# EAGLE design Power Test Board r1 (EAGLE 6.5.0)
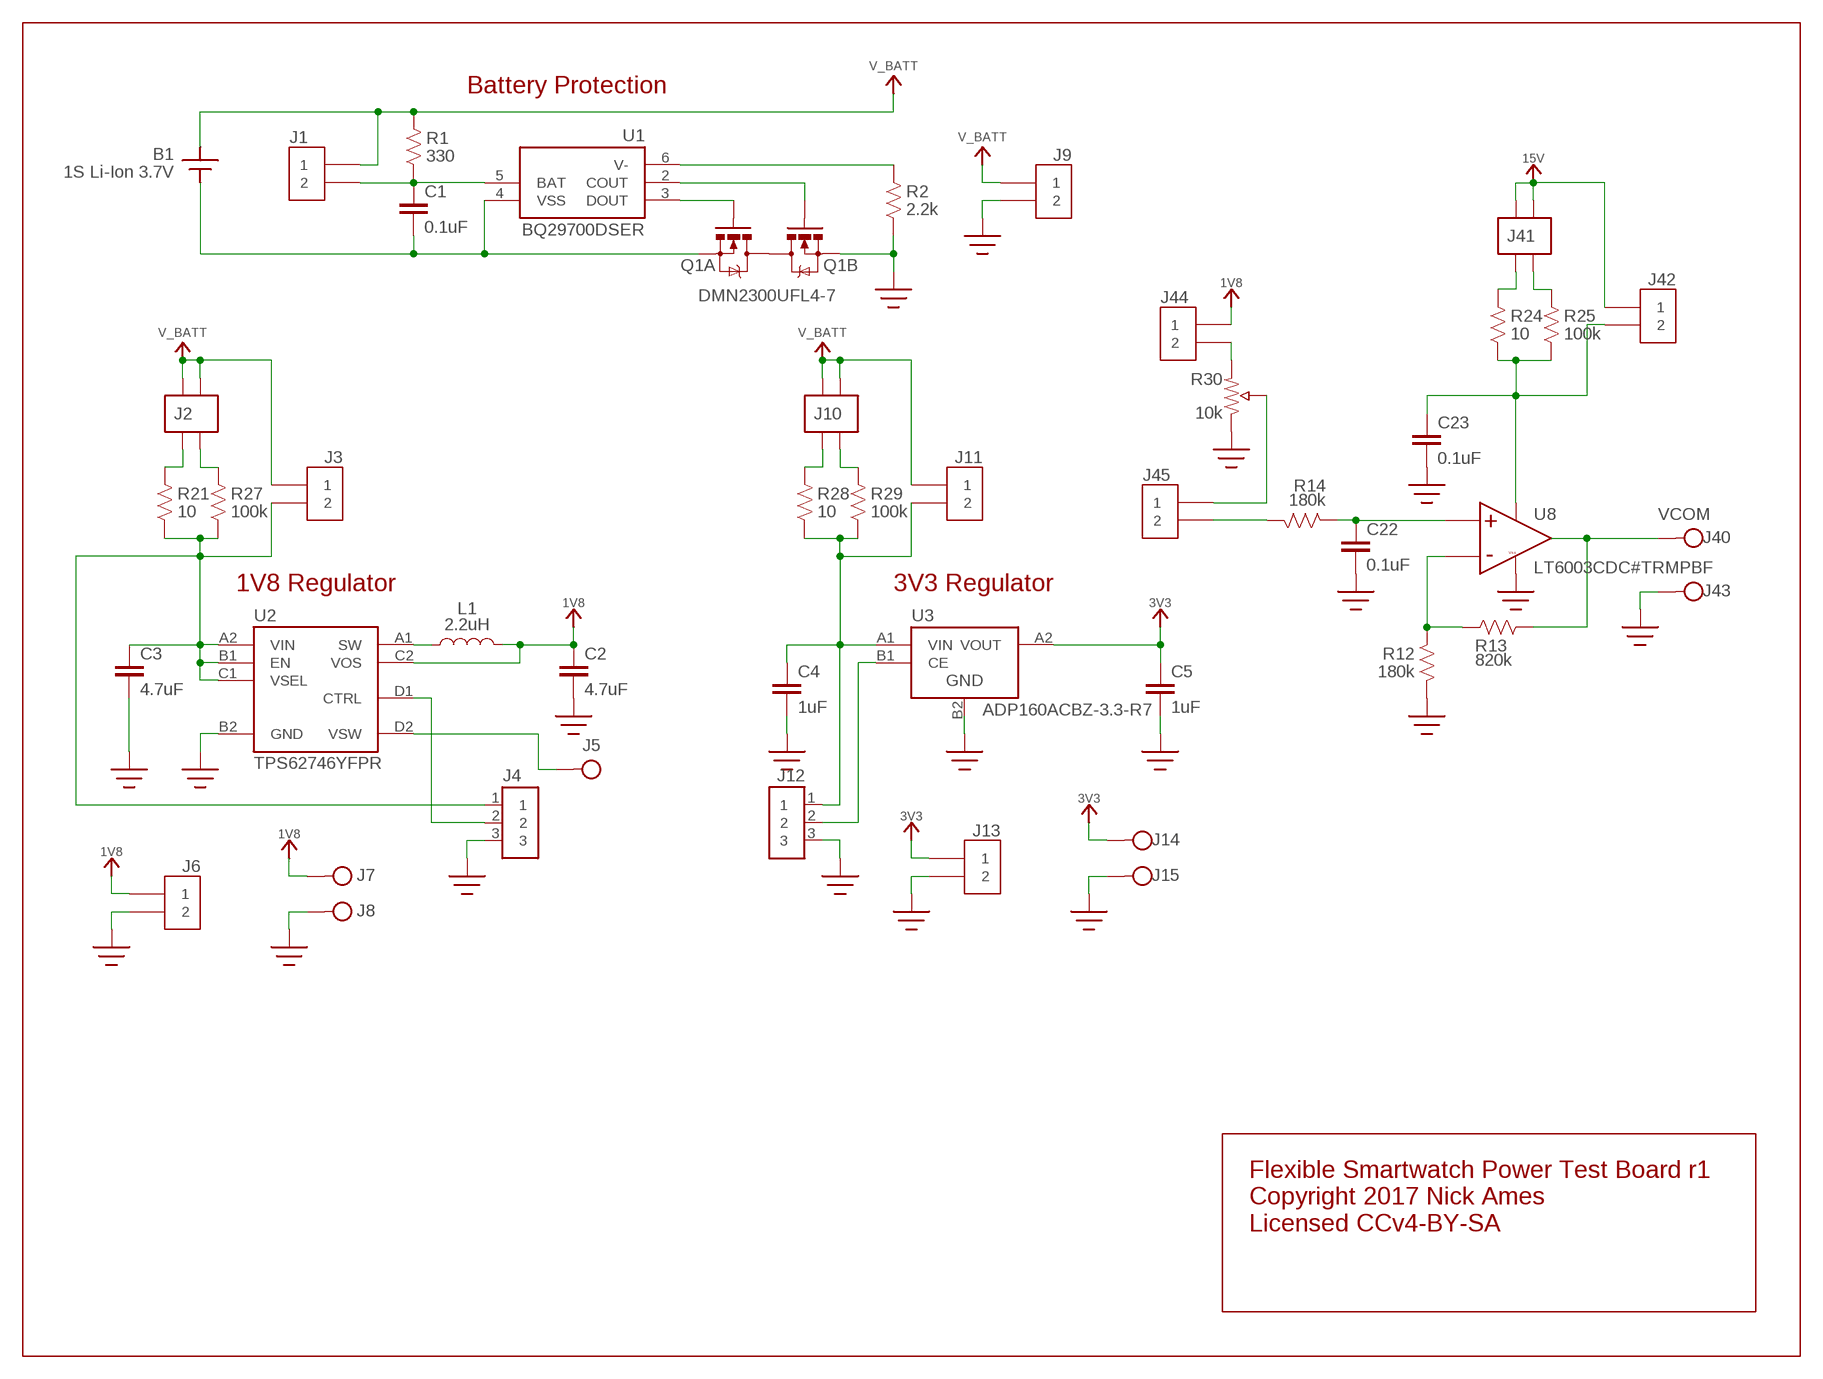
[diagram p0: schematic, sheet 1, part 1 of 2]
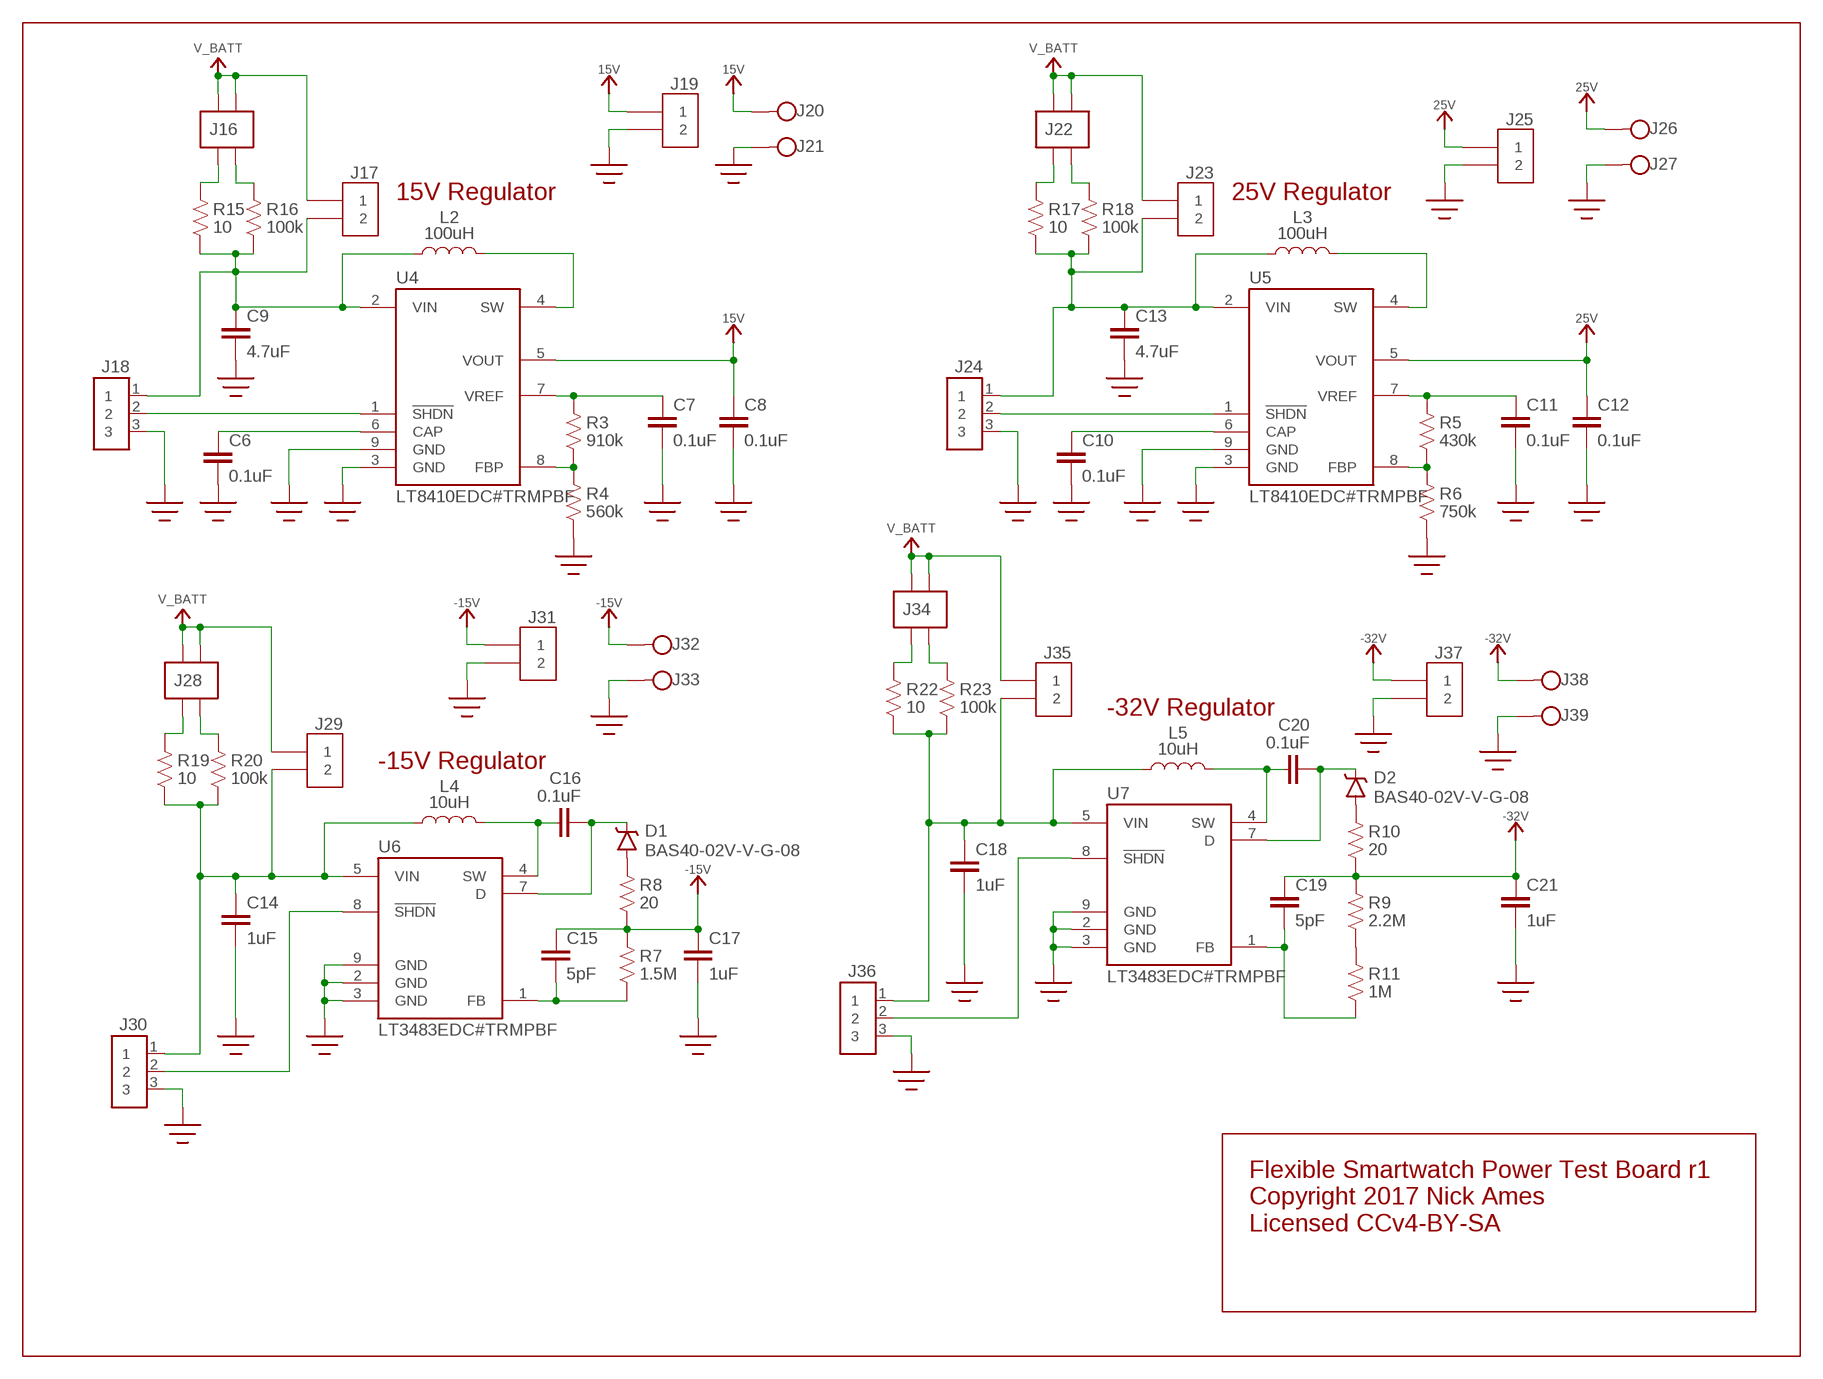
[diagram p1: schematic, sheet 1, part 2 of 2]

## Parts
B1  1S Li-Ion 3.7V  BATTERY-1CELLWIRE_TERMINAL_PTH  [BATTERY-WIRETERM]
C1  0.1uF  CAP201  [0201]
C2  4.7uF  CAP201  [0201]
C3  4.7uF  CAP201  [0201]
C4  1uF  CAP201  [0201]
C5  1uF  CAP201  [0201]
C6  0.1uF  CAP201  [0201]
C7  0.1uF  CAP201  [0201]
C8  0.1uF  CAP201  [0201]
C9  4.7uF  CAP201  [0201]
C10  0.1uF  CAP201  [0201]
C11  0.1uF  CAP201  [0201]
C12  0.1uF  CAP201  [0201]
C13  4.7uF  CAP201  [0201]
C14  1uF  CAP201  [0201]
C15  5pF  CAP201  [0201]
C16  0.1uF  CAP201  [0201]
C17  1uF  CAP402  [0402]
C18  1uF  CAP201  [0201]
C19  5pF  CAP201  [0201]
C20  0.1uF  CAP201  [0201]
C21  1uF  CAP402  [0402]
C22  0.1uF  CAP201  [0201]
C23  0.1uF  CAP201  [0201]
D1  BAS40-02V-V-G-08  DIODE-SCHOTTKYSOD-523  [SOD-523]
D2  BAS40-02V-V-G-08  DIODE-SCHOTTKYSOD-523  [SOD-523]
J1  HEADER-02HEADER-02  [HEADER-02]
J2  HEADER-02X02  [HEADER-02X02]
J3  HEADER-02HEADER-02  [HEADER-02]
J4  HEADER-03PTH  [HEADER-03]
J5  TESTPOINTPTH  [TESTPOINT-1-PTH]
J6  HEADER-02HEADER-02  [HEADER-02]
J7  TESTPOINTPTH  [TESTPOINT-1-PTH]
J8  TESTPOINTPTH  [TESTPOINT-1-PTH]
J9  HEADER-02HEADER-02  [HEADER-02]
J10  HEADER-02X02  [HEADER-02X02]
J11  HEADER-02HEADER-02  [HEADER-02]
J12  HEADER-03PTH  [HEADER-03]
J13  HEADER-02HEADER-02  [HEADER-02]
J14  TESTPOINTPTH  [TESTPOINT-1-PTH]
J15  TESTPOINTPTH  [TESTPOINT-1-PTH]
J16  HEADER-02X02  [HEADER-02X02]
J17  HEADER-02HEADER-02  [HEADER-02]
J18  HEADER-03PTH  [HEADER-03]
J19  HEADER-02HEADER-02  [HEADER-02]
J20  TESTPOINTPTH  [TESTPOINT-1-PTH]
J21  TESTPOINTPTH  [TESTPOINT-1-PTH]
J22  HEADER-02X02  [HEADER-02X02]
J23  HEADER-02HEADER-02  [HEADER-02]
J24  HEADER-03PTH  [HEADER-03]
J25  HEADER-02HEADER-02  [HEADER-02]
J26  TESTPOINTPTH  [TESTPOINT-1-PTH]
J27  TESTPOINTPTH  [TESTPOINT-1-PTH]
J28  HEADER-02X02  [HEADER-02X02]
J29  HEADER-02HEADER-02  [HEADER-02]
J30  HEADER-03PTH  [HEADER-03]
J31  HEADER-02HEADER-02  [HEADER-02]
J32  TESTPOINTPTH  [TESTPOINT-1-PTH]
J33  TESTPOINTPTH  [TESTPOINT-1-PTH]
J34  HEADER-02X02  [HEADER-02X02]
J35  HEADER-02HEADER-02  [HEADER-02]
J36  HEADER-03PTH  [HEADER-03]
J37  HEADER-02HEADER-02  [HEADER-02]
J38  TESTPOINTPTH  [TESTPOINT-1-PTH]
J39  TESTPOINTPTH  [TESTPOINT-1-PTH]
J40  TESTPOINTPTH  [TESTPOINT-1-PTH]
J41  HEADER-02X02  [HEADER-02X02]
J42  HEADER-02HEADER-02  [HEADER-02]
J43  TESTPOINTPTH  [TESTPOINT-1-PTH]
J44  HEADER-02HEADER-02  [HEADER-02]
J45  HEADER-02HEADER-02  [HEADER-02]
L1  2.2uH  INDUCTOR603  [0603-RES]
L2  100uH  INDUCTOR805  [0805-IND]
L3  100uH  INDUCTOR805  [0805-IND]
L4  10uH  INDUCTORMDKK2020  [TY_MDKK2020]
L5  10uH  INDUCTORMDKK2020  [TY_MDKK2020]
Q1  DMN2300UFL4-7  MOSFET-N-DUALDFN  [DFN1310-6]
R1  330  RESISTOR201  [0201]
R2  2.2k  RESISTOR201  [0201]
R3  910k  RESISTOR201  [0201]
R4  560k  RESISTOR201  [0201]
R5  430k  RESISTOR201  [0201]
R6  750k  RESISTOR201  [0201]
R7  1.5M  RESISTOR201  [0201]
R8  20  RESISTOR201  [0201]
R9  2.2M  RESISTOR201  [0201]
R10  20  RESISTOR201  [0201]
R11  1M  RESISTOR201  [0201]
R12  180k  RESISTOR201  [0201]
R13  820k  RESISTOR201  [0201]
R14  180k  RESISTOR201  [0201]
R15  10  RESISTOR0603-RES  [0603-RES]
R16  100k  RESISTOR0603-RES  [0603-RES]
R17  10  RESISTOR0603-RES  [0603-RES]
R18  100k  RESISTOR0603-RES  [0603-RES]
R19  10  RESISTOR0603-RES  [0603-RES]
R20  100k  RESISTOR0603-RES  [0603-RES]
R21  10  RESISTOR0603-RES  [0603-RES]
R22  10  RESISTOR0603-RES  [0603-RES]
R23  100k  RESISTOR0603-RES  [0603-RES]
R24  10  RESISTOR0603-RES  [0603-RES]
R25  100k  RESISTOR0603-RES  [0603-RES]
R27  100k  RESISTOR0603-RES  [0603-RES]
R28  10  RESISTOR0603-RES  [0603-RES]
R29  100k  RESISTOR0603-RES  [0603-RES]
R30  10k  POTPVZA3  [PVZ3A]
U1  BQ29700DSER  TI-BQ29700_BATTERY_PROTECTOR  [6-SON_TI_DSE]
U2  TPS62746YFPR  TI-TPS62746_VREG_BUCK_VSWITCH  [8-XBGA_TI_YFP]
U3  ADP160ACBZ-3.3-R7  AD_ADP160CBZ  [WLCSP-4-.5]
U4  LT8410EDC#TRMPBF  LT-LT8410_VREG_BOOST  [8-DFN_LT_DC]
U5  LT8410EDC#TRMPBF  LT-LT8410_VREG_BOOST  [8-DFN_LT_DC]
U6  LT3483EDC#TRMPBF  LT-LT3483_VREG_INVERT  [8-DFN_LT_DC]
U7  LT3483EDC#TRMPBF  LT-LT3483_VREG_INVERT  [8-DFN_LT_DC]
U8  LT6003CDC#TRMPBF  OPAMPLT6003  [DFN-4_LT_DC]

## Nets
1V8: C2.P$1 J6.1 J7.1 J44.1 L1.2 U2.C2(VOS)
3V3: C5.P$1 J13.1 J14.1 U3.A2(VOUT)
15V: C8.P$1 J19.1 J20.1 J41.1 J41.4 J42.1 U4.5(VOUT)
25V: C12.P$1 J25.1 J26.1 U5.5(VOUT)
-15V: C15.P$1 C17.1 J31.1 J32.1 R7.P$2 R8.P$1
-32V: C19.P$1 C21.1 J37.1 J38.1 R9.P$2 R10.P$1
GND: C2.P$2 C3.P$2 C4.P$2 C5.P$2 C6.P$2 C7.P$2 C8.P$2 C9.P$2 C10.P$2 C11.P$2 C12.P$2 C13.P$2 C14.P$2 C17.2 C18.P$2 C21.2 C22.P$2 C23.P$2 J4.3 J6.2 J8.1 J9.2 J12.3 J13.2 J15.1 J18.3 J19.2 J21.1 J24.3 J25.2 J27.1 J30.3 J31.2 J33.1 J36.3 J37.2 J39.1 J43.1 Q1.S2(B:S) R2.P$1 R4.P$1 R6.P$1 R12.P$1 R30.1(A) U2.B2(GND) U3.B2(GND) U4.3(GND) U4.9(GND) U5.3(GND) U5.9(GND) U6.2(GND) U6.3(GND) U6.9(GND) U7.2(GND) U7.3(GND) U7.9(GND) U8.5(VSS)
N$1: C1.P$1 J1.2 R1.P$1 U1.5(BAT)
N$2: B1.- C1.P$2 Q1.S1(A:S) U1.4(VSS)
N$3: C3.P$1 J3.2 J4.1 R21.1 R27.1 U2.A2(VIN) U2.B1(EN) U2.C1(VSEL)
N$4: Q1.D1(A:D) Q1.D2(B:D)
N$5: Q1.G1(A:G) U1.3(DOUT)
N$6: Q1.G2(B:G) U1.2(COUT)
N$7: R2.P$2 U1.6(V-)
N$8: L1.1 U2.A1(SW)
N$9: C14.P$1 J29.2 J30.1 L4.1 R19.1 R20.1 U6.5(VIN)
N$10: J12.2 U3.B1(CE)
N$11: C4.P$1 J11.2 J12.1 R28.1 R29.1 U3.A1(VIN)
N$12: J10.3 R28.2
N$13: C6.P$1 U4.6(CAP)
N$14: J18.2 U4.1(!SHDN!)
N$15: C9.P$1 J17.2 J18.1 L2.P$1 R15.1 R16.1 U4.2(VIN)
N$16: C7.P$1 R3.P$2 U4.7(VREF)
N$17: L2.P$2 U4.4(SW)
N$18: R3.P$1 R4.P$2 U4.8(FBP)
N$19: C10.P$1 U5.6(CAP)
N$20: J24.2 U5.1(!SHDN!)
N$21: J30.2 U6.8(!SHDN!)
N$22: C11.P$1 R5.P$2 U5.7(VREF)
N$23: L3.P$2 U5.4(SW)
N$24: R5.P$1 R6.P$2 U5.8(FBP)
N$25: J2.3 R21.2
N$26: J2.2 R27.2
N$27: J10.2 R29.2
N$28: J4.2 U2.D1(CTRL)
N$29: J5.1 U2.D2(VSW)
N$30: J16.3 R15.2
N$31: J16.2 R16.2
N$32: C13.P$1 J23.2 J24.1 L3.P$1 R17.1 R18.1 U5.2(VIN)
N$33: C16.P$1 L4.2 U6.4(SW)
N$34: D1.A R8.P$2
N$35: C16.P$2 D1.C U6.7(D)
N$36: J22.3 R17.2
N$37: J22.2 R18.2
N$38: C23.P$1 J42.2 R24.1 R25.1 U8.4(VDD)
N$39: C15.P$2 R7.P$1 U6.1(FB)
N$40: J36.2 U7.8(!SHDN!)
N$41: C20.P$1 L5.2 U7.4(SW)
N$42: D2.A R10.P$2
N$43: C20.P$2 D2.C U7.7(D)
N$44: C19.P$2 R11.P$1 U7.1(FB)
N$45: J34.3 R22.2
N$46: R9.P$1 R11.P$2
N$47: J28.3 R19.2
N$48: J28.2 R20.2
N$49: J34.2 R23.2
N$50: C18.P$1 J35.2 J36.1 L5.1 R22.1 R23.1 U7.5(VIN)
N$51: J41.3 R24.2
N$52: R12.P$2 R13.P$1 U8.2(-)
N$53: C22.P$1 R14.P$1 U8.1(+)
N$54: J44.2 R30.3(E)
N$55: J41.2 R25.2
N$57: J45.2 R14.P$2
N$58: J45.1 R30.2(S)
V_BATT: B1.+ J1.1 J2.1 J2.4 J3.1 J9.1 J10.1 J10.4 J11.1 J16.1 J16.4 J17.1 J22.1 J22.4 J23.1 J28.1 J28.4 J29.1 J34.1 J34.4 J35.1 R1.P$2
VCOM: J40.1 R13.P$2 U8.3(OUT)

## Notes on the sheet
- Battery Protection
- 15V Regulator | 25V Regulator
- 1V8 Regulator | 3V3 Regulator
- -32V Regulator
- -15V Regulator
- Flexible Smartwatch Power Test Board r1
  Copyright 2017 Nick Ames
  Licensed CCv4-BY-SA
- Flexible Smartwatch Power Test Board r1
  Copyright 2017 Nick Ames
  Licensed CCv4-BY-SA

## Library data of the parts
B1 = NA-lib:BATTERY-1CELL
C1-C23 = NA-lib:CAP: Capacitor
D1 D2 = NA-lib:DIODE-SCHOTTKY
J1 J3 J6 J9 J11 J13 J17 J19 J23 J25 J29 J31 J35 J37 J42 J44 J45 = NA-lib:HEADER-02
J2 J10 J16 J22 J28 J34 J41 = NA-lib:HEADER-02X02
J4 J12 J18 J24 J30 J36 = NA-lib:HEADER-03
J5 J7 J8 J14 J15 J20 J21 J26 J27 J32 J33 J38-J40 J43 = NA-lib:TESTPOINT
L1-L5 = NA-lib:INDUCTOR: Inductors
Q1 = NA-lib:MOSFET-N-DUAL
R1-R25 R27-R29 = NA-lib:RESISTOR: Resistor
R30 = NA-lib:POT
U1 = Project-6p:TI-BQ29700_BATTERY_PROTECTOR
U2 = Project-6p:TI-TPS62746_VREG_BUCK_VSWITCH
U3 = NA-lib:AD_ADP160
U4 U5 = Project-6p:LT-LT8410_VREG_BOOST
U6 U7 = Project-6p:LT-LT3483_VREG_INVERT
U8 = NA-lib:OPAMP

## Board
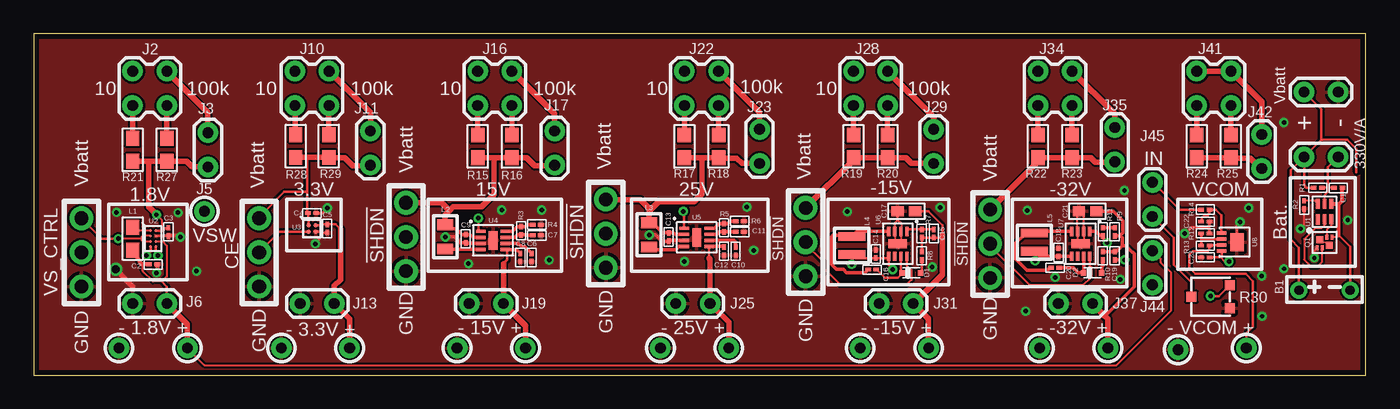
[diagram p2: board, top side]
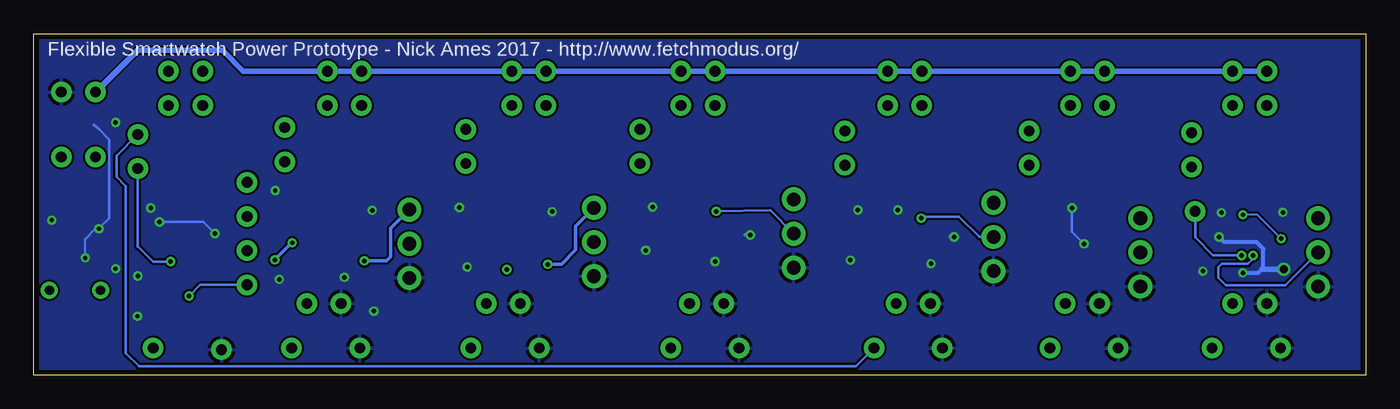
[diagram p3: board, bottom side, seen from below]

Size 99.06 x 25.4 mm. Coordinates in mm from the lower left corner, seen from the top.
Outline: 0,0 99.06,0 99.06,25.4 0,25.4 0,0
Copper layers (1*16): Top 0.0356mm / dielectric 1.5011mm / Bottom 0.0356mm
Design rules "LaenPCBOrder-tented_vias": minimum track width 6mil, minimum drill 13mil, track to track 6mil, track to pad 6mil, pad to pad 6mil, via to via 6mil, smd to smd 6mil, copper to edge 15mil, drill to drill 6mil, minimum pad ring 7mil, minimum via ring 7mil, stop-mask expansion 3mil, vias tented up to drill 25mil, thermal gap 10mil
tRestrict: area 63.8,10.2 to 64.8,11.7; area 77.3,10.2 to 78.4,11.7

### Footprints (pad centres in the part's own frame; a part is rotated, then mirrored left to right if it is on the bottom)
BATTERY-WIRETERM = drill 0.7 pad 1.27: + -1.905,0; - 1.905,0
0201 = smd 0.406 x 0.279: P$1 -0.305,0; P$2 0.305,0
0402 = smd 0.9 x 0.762: 1 -0.65,0; 2 0.65,0
SOD-523 = smd 0.406 x 0.406: A 0.686,0; C -0.686,0
HEADER-02 = drill 0.8 pad 1.524: 1 -1.27,0; 2 1.27,0
HEADER-02X02 = drill 0.8 pad 1.524: 1 1.27,1.27; 2 1.27,-1.27; 3 -1.27,-1.27; 4 -1.27,1.27
HEADER-03 = drill 1.016 pad 1.778: 1 0,2.54; 2 0,0; 3 0,-2.54
TESTPOINT-1-PTH = drill 0.8 pad 1.524: 1 0,0
0603-RES = smd 1.1 x 1: 1 -0.85,0; 2 0.85,0
0805-IND = smd 0.8 x 1.2: P$1 -0.9,0; P$2 0.9,0
TY_MDKK2020 = smd 0.65 x 2: 1 -0.675,0; 2 0.675,0
DFN1310-6 = smd 0.51 x 0.51: D1 -0.35,0.2; D2 0.35,-0.2 | smd 0.2 x 0.375: G1 -0.17,-0.4; G2 0.17,0.4; S1 -0.55,-0.4; S2 0.55,0.4
PVZ3A = smd 0.75 x 0.75: 1 -0.85,-1.425; 2 0,1.425; 3 0.85,-1.425
6-SON_TI_DSE = smd 0.78 x 0.28: 1 -0.57,0.5 | smd 0.75 x 0.28: 2 -0.575,0; 3 -0.575,-0.5; 4 0.575,-0.5; 5 0.575,0; 6 0.575,0.5
8-XBGA_TI_YFP = smd 0.23 x 0.23: A1 -0.2,0.6; A2 0.2,0.6; B1 -0.2,0.2; B2 0.2,0.2; C1 -0.2,-0.2; C2 0.2,-0.2; D1 -0.2,-0.6; D2 0.2,-0.6
WLCSP-4-.5 = smd 0.32 x 0.32: A1 -0.25,0.25; A2 0.25,0.25; B1 -0.25,-0.25; B2 0.25,-0.25
8-DFN_LT_DC = smd 0.25 x 0.7: 1 -0.675,-0.925; 2 -0.225,-0.925; 3 0.225,-0.925; 4 0.675,-0.925; 5 0.675,0.925; 6 0.225,0.925; 7 -0.225,0.925; 8 -0.675,0.925 | smd 1.37 x 0.64: 9 0,0
DFN-4_LT_DC = smd 0.25 x 0.7: 1 -0.675,-0.95; 2 -0.225,-0.95; 3 0.225,-0.95; 4 0.675,-0.95 | smd 1.35 x 1: 5 0,0.2

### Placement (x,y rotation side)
B1  95.99,6.32 0 top
C1  97,13.94 0 top
C2  8.89,8.26 0 top
C3  10.03,10.67 270 top
C4  20.7,12.06 0 top
C5  21.84,10.92 270 top
C6  37.03,8.76 270 top
C7  37.41,10.41 0 top
C8  36.2,8.76 270 top
C9  32.13,10.16 270 top
C10  52.2,9.22 270 top
C11  52.5,10.67 0 top
C12  51.33,9.22 270 top
C13  47.22,10.29 270 top
C14  62.61,9.02 90 top
C15  66.93,10.54 90 top
C16  62.36,7.87 0 top
C17  64.9,12.19 180 top
C18  76.2,9.14 90 top
C19  80.39,8.89 270 top
C20  75.95,8 0 top
C21  78.36,12.19 180 top
C22  87.12,11.43 0 top
C23  87.12,8.76 180 top
D1  65.28,7.62 0 top
D2  78.74,7.62 0 top
J1  95.73,16.23 0 top
J2  8.64,21.34 0 top
J3  12.95,16.76 270 top
J4  3.56,9.14 0 top
J5  12.7,12.19 0 top
J6  8.64,5.33 180 top
J7  11.43,2.03 0 top
J8  6.35,2.03 0 top
J9  95.73,21.06 0 top
J10  20.7,21.34 0 top
J11  25.04,16.89 270 top
J12  16.76,9.14 0 top
J13  21.08,5.33 180 top
J14  23.5,2.03 0 top
J15  18.41,2.03 0 top
J16  34.29,21.34 0 top
J17  38.73,16.89 270 top
J18  27.69,10.29 0 top
J19  33.66,5.33 180 top
J20  36.58,2.03 0 top
J21  31.5,2.03 0 top
J22  49.66,21.34 0 top
J23  53.98,17.02 270 top
J24  42.55,10.54 0 top
J25  49.02,5.33 180 top
J26  51.69,2.03 0 top
J27  46.61,2.03 0 top
J28  62.23,21.34 0 top
J29  66.93,17.02 270 top
J30  57.4,9.91 0 top
J31  64.14,5.33 180 top
J32  66.55,2.03 0 top
J33  61.47,2.03 0 top
J34  75.95,21.34 0 top
J35  80.39,17.14 270 top
J36  71.12,9.78 0 top
J37  77.47,5.33 180 top
J38  79.88,2.03 0 top
J39  74.8,2.03 0 top
J40  90.17,2.03 0 top
J41  87.76,21.34 0 top
J42  91.31,16.64 270 top
J43  85.09,1.91 0 top
J44  83.19,8 270 top
J45  83.19,13.08 90 top
L1  7.37,10.16 270 top
L2  30.61,10.29 270 top
L3  45.75,10.44 270 top
L4  60.83,9.65 90 top
L5  74.42,9.91 90 top
Q1  95.99,9.88 180 top
R1  95.48,13.94 180 top
R2  94.46,12.67 90 top
R3  36.25,10.74 270 top
R4  37.41,11.2 180 top
R5  51.33,10.97 270 top
R6  52.5,11.46 180 top
R7  66.04,10.54 270 top
R8  66.04,8.89 270 top
R9  80.39,10.67 270 top
R10  79.5,8.89 270 top
R11  79.5,10.67 90 top
R12  87.12,10.54 180 top
R13  87.12,9.65 0 top
R14  87.12,12.32 180 top
R15  33.02,17.02 90 top
R16  35.56,17.02 90 top
R17  48.39,17.02 90 top
R18  50.93,17.02 90 top
R19  60.96,17.02 90 top
R20  63.5,17.02 90 top
R21  7.37,16.76 90 top
R22  74.68,17.02 90 top
R23  77.22,17.02 90 top
R24  86.49,17.02 90 top
R25  89.03,17.02 90 top
R27  9.91,16.76 90 top
R28  19.48,17.04 90 top
R29  21.95,17.04 90 top
R30  87.5,5.84 90 top
U1  95.99,12.17 90 top
U2  8.89,10.16 0 top
U3  20.7,10.92 0 top
U4  34.16,10.03 270 top
U5  49.3,10.26 270 top
U6  64.26,9.78 180 top
U7  77.85,9.78 180 top
U8  89.28,9.91 270 top

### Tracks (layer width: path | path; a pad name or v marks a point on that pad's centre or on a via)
1V8
  Top 0.152: U2.C2 9.6,9.96 9.91,9.65 9.91,7.37 9.53,6.99 8.89,6.99 8.13,7.75 8.13,8.26 | J7.1 12.7,0.76 80.52,0.76 84.58,4.83 84.58,7.62 83.82,8.38 83.82,8.64 J44.1
  Top 0.203: J6.1 9.91,6.6 9.53,6.99
  Top 0.305: C2.P$1 8.13,8.26 8,8.26 7.62,8.89 L1.2
  Top 0.406: J7.1 11.43,3.81 J6.1
3V3
  Top 0.203: U3.A2 21.46,11.18 21.51,11.23 C5.P$1 22.45,11.23 22.81,10.87
  Top 0.406: 22.81,10.87 22.81,7.11 22.35,6.66 22.35,5.51 22.33,5.49 22.33,5.36 J13.1 23.5,4.19 J14.1
15V
  Top 0.203: 35.2,9.35 35.2,8.59 34.92,8.31
  Top 0.254: C8.P$1 35.92,9.35 35.2,9.35 35.1,9.35 U4.5
  Top 0.406: J41.4 J41.1 91.31,20.32 J42.1 | 34.92,8.31 J19.1 36.58,3.68 J20.1
  Bottom 0.203: J20.1 36.58,2.01 37.92,0.66 91.21,0.66 92.2,1.65 92.2,14.07 92.89,14.76 92.89,16.33 J42.1
25V
  Top 0.203: U5.5 50.22,9.58 50.22,8.71
  Top 0.254: U5.5 51.27,9.59 C12.P$1
  Top 0.406: J26.1 51.69,3.94 J25.1 50.29,8.64 50.22,8.71
-15V
  Top 0.203: R8.P$1 R7.P$2 C15.P$1 67.39,10.24 67.56,10.41 67.56,11.18 66.55,12.19 C17.1
  Top 0.406: J32.1 66.55,4.19 J31.1 67.56,7.49 67.56,10.41
-32V
  Top 0.254: C21.1 80.29,12.19 81,11.48 81,10.62 80.77,10.39 | 80.77,10.39 80.42,10.39 R9.P$2 | R10.P$1 C19.P$1 80.49,9.2 80.95,9.65 | 80.95,9.65 80.95,10.21 80.77,10.39 | 80.95,9.65 81.2,9.65 81.71,9.14 81.74,9.14 81.84,9.04 81.84,6.58 79.67,4.41
  Top 0.406: J37.1 79.67,4.41 79.88,4.19 J38.1
GND  (via drill 0.33 pad 0.69, 0.6 pad 0.69)
  Top 0.152: Q1.S2 95.22,9.27 v95.22,8.74 | v94.21,10.9 94.46,11.15 R2.P$1 | C3.P$2 | C17.2 64.25,11.54 | 64.25,11.54 64.01,11.3 64.01,10.73 U6.3 64.04,9.81 64.01,9.78 U6.9 64.49,10 U6.2 64.52,10.73 64.52,11.3 64.28,11.54 64.25,11.54 | 77.6,9.78 77.63,9.81 U7.3 77.63,12.11 C21.2 78.08,11.82 U7.2 78.08,9.81 78.11,9.78
  Top 0.203: U2.B2 C3.P$2 | U3.B2 21.46,10.67 21.51,10.62 | 21.51,10.62 C5.P$2 | C4.P$2 21.46,12.06 v21.84,12.45 | v20.95,9.78 21.34,10.29 21.34,10.57 21.51,10.62 | 87.43,11 86.13,11 85.67,10.54 v85.57,10.54 | v89.71,11.4 89.48,11.17 U8.5 | R12.P$1 87.43,11 | 87.43,11 C22.P$2 | C23.P$2 86.84,8.74
  Top 0.254: U4.3 32.18,9.81 C9.P$2 31.75,9.86 31.32,10.29 v30.61,10.29 | U5.3 47.27,10.04 C13.P$2 46.71,9.98 46.25,10.44 v45.77,10.44
  Top 0.305: C2.P$2 9.2,7.67 v9.14,7.62 | v10.92,10.29 10.85,10.36 C3.P$2
  Top 0.406: 7.37,6.6 v6.1,7.87
  Bottom 0.152: v95.22,8.74 95.22,10.13 94.46,10.9 v94.21,10.9
  Bottom 0.203: v21.84,12.45 21.84,10.67 v20.95,9.78 | v94.21,10.9 94.21,10.92 93.45,11.68 93.45,17.53 94.23,18.31 94.59,18.64 | v85.57,10.54 86.44,11.4 v89.71,11.4
  Bottom 0.254: v30.61,10.29 30.91,10.29 | v45.77,10.44 46.18,10.44
  Bottom 0.305: v9.14,7.62 8,7.62 7.68,7.94 7.62,8 7.62,9.4 8.13,9.91 10.54,9.91 v10.92,10.29
  Bottom 0.406: v6.1,7.87 7.62,7.87 7.68,7.94
  other vias: 60.5,12.17 53.04,12.52 53.54,9.3 48.39,8.46 67.41,12.47 66.83,8.05 73.89,12.27 81.1,13.74 75.95,7.29 80.8,7.14 73.76,4.78 37.77,12.29 34.8,12.29 32.33,8.31 38.33,8.56 10.74,12.09 6.17,12.12 12.12,7.75 97.71,11.53 90.35,12.45 91.31,7.39 91.34,4.39 92.96,18.8 92.96,7.92
  pour Bottom: 0,0 99.06,0 99.06,25.4 0,25.4
  pour Top: 0,0 99.06,0 99.06,25.4 0,25.4
N$1
  Top 0.152: 95.78,13.89 R1.P$1 96.24,13.95 | C1.P$1 96.24,13.95 | U1.5 95.99,13.39 96.24,13.64 96.24,13.95
  Top 0.203: 96.24,13.95 96.24,15.47 J1.2
N$2
  Top 0.152: 97,10.39 96.89,10.28 Q1.S1
  Top 0.203: B1.- 97.89,9.55 97,10.44
  Top 0.305: U1.4 97.07,12.74 | 97.07,12.74 97.31,12.98 C1.P$2 | 97.07,12.74 97,12.68 97,10.44 97,10.39
N$3  (via drill 0.33 pad 0.69)
  Top 0.152: 9.98,10.92 C3.P$1 | U2.B1 8.12,10.36 8.05,10.29 8.05,10.16 | U2.C1 8.12,9.96 8.05,10.03 8.05,10.16 | 8.05,10.16 v6.3,10.16 | v9.14,11.94 9.53,11.56 9.53,11.05 9.72,10.86
  Top 0.203: U2.A2 9.62,10.76 9.72,10.86 9.78,10.92 9.98,10.92 | J4.1 5.08,10.16 v6.3,10.16
  Top 0.406: R21.1 8.54,15.91 | 8.54,15.91 R27.1 11.37,15.91 11.79,15.49 J3.2 | 8.54,15.91 8.54,12.54 v9.14,11.94
  Bottom 0.152: v6.3,10.16 8.08,11.94 v9.14,11.94
N$4
  Top 0.152: Q1.D2 95.81,9.91 | Q1.D2 95.66,9.91 | Q1.D1 96.39,9.68 96.52,9.86 95.48,9.91 95.63,10.08 Q1.D2
N$5
  Top 0.152: U1.3 96.5,11.15 96.16,10.81 Q1.G1
N$6
  Top 0.152: U1.2 95.99,11.2 95.73,10.95 95.3,10.95 94.46,10.13 94.46,8.61 94.97,8.1 95.48,8.1 95.82,8.44 Q1.G2
N$7
  Top 0.152: U1.6 95.25,12.98 R2.P$2
N$8
  Top 0.152: U2.A1 7.62,10.76 L1.1
N$9  (via drill 0.33 pad 0.69)
  Top 0.203: v63.88,7.87 63.59,8.17 U6.5 63.45,8.71 C14.P$1 61.1,8.71 L4.1
  Top 0.254: L4.1 v60.83,8.26
  Top 0.406: J29.2 65.28,15.75 64.86,16.17 R20.1 R19.1 60.96,16 J30.1
  Bottom 0.254: v60.83,8.26 59.82,8.26 58.75,9.32 58.75,11.1 J30.1
N$10
  Top 0.203: U3.B1 18.29,10.67 J12.2
N$11
  Top 0.152: R29.1 22.46,16.19 22.48,16.18
  Top 0.203: U3.A1 20.45,11.68 20.4,11.73 C4.P$1 20.32,12.14 20.32,13.61 | 21.91,16.19 22.1,16 | 20.32,13.61 20.32,16.17 20.3,16.19 | J12.1 16.76,11.76 18.64,13.64 20.3,13.64 20.32,13.61
  Top 0.406: R28.1 20.3,16.19 21.91,16.19 R29.1 22.09,16.19 22.1,16.2 22.12,16.2 22.15,16.18 22.48,16.18 23.14,16.18 23.72,15.6 25.02,15.6 J11.2
N$12
  Top 0.406: J10.3 19.43,17.94 R28.2
N$13
  Top 0.254: U4.6 36.04,9.81 36.27,9.58 36.52,9.58 C6.P$1
N$14  (via drill 0.33 pad 0.69)
  Top 0.203: v33.07,11.68 33.07,10.72 33.23,10.72 U4.1
  Bottom 0.203: J18.2 28.75,10.29 30.25,11.79 32.97,11.79 v33.07,11.68
N$15
  Top 0.254: U4.2 32.67,10.26 32.46,10.46 C9.P$1 31.85,10.46 31.42,10.9 30.94,10.9 30.91,10.92 30.87,10.92 L2.P$1
  Top 0.406: R15.1 34.24,16.17 | 34.24,16.17 R16.1 36.66,16.17 37.24,15.6 38.71,15.6 J17.2 | 34.24,16.17 34.24,13.47 33.3,12.52 31.19,12.52 30.91,12.24 | 30.91,12.24 30.61,11.94 L2.P$1 | J18.1 30.33,12.83 30.91,12.24
N$16
  Top 0.254: U4.7 35.81,10.26 35.99,10.44 R3.P$2 36.68,10.44 36.7,10.41 C7.P$1
N$17
  Top 0.254: U4.4 30.64,9.36 L2.P$2
N$18
  Top 0.254: U4.8 35.6,10.71 35.94,11.05 R3.P$1 36.55,11.05 36.7,11.2 R4.P$2
N$19
  Top 0.254: U5.6 52.09,10.04 52.2,9.93 C10.P$1
N$20  (via drill 0.33 pad 0.69)
  Top 0.203: v48.31,12.19 48.38,12.2 U5.1
  Bottom 0.203: J24.2 44.27,12.27 v48.31,12.19
N$21
  Top 0.203: J30.2 57.4,9.75 58.67,8.48 58.67,8.03 59.94,6.76 64.92,6.76 65.28,7.11 65.28,7.8 64.92,8.15 64.92,8.84 U6.8
N$22
  Top 0.254: U5.7 50.8,10.49 50.98,10.67 R5.P$2 C11.P$1
N$23
  Top 0.254: U5.4 47.99,9.59 47.75,9.35 46.05,9.35 45.87,9.53 45.76,9.53 L3.P$2
N$24
  Top 0.254: U5.8 50.61,10.94 50.95,11.28 R5.P$1 51.59,11.28 51.77,11.46 R6.P$2
N$25
  Top 0.406: J2.3 R21.2
N$26
  Top 0.406: J2.2 R27.2
N$27
  Top 0.406: R29.2 21.95,20.04 J10.2
N$28  (via drill 0.33 pad 0.69)
  Top 0.203: U2.D1 8.69,9.22 v8.38,8.91
  Bottom 0.203: J4.2 5.99,6.71 10.41,6.71 10.97,7.26 10.97,8.03 10.72,8.28 8.76,8.28 8.38,8.66 v8.38,8.91
N$29  (via drill 0.33 pad 0.69)
  Top 0.203: U2.D2 9.09,9.07 v9.25,8.91
  Bottom 0.203: J5.1 12.7,10.26 11.38,8.94 9.27,8.94 v9.25,8.91
N$30
  Top 0.406: J16.3 R15.2
N$31
  Top 0.406: J16.2 R16.2
N$32
  Top 0.254: U5.2 47.7,10.49 47.57,10.62 47.24,10.62 C13.P$1 46.76,10.59 46.08,11.28 45.81,11.28 L3.P$1
  Top 0.406: R17.1 49.69,16.17 | 49.69,16.17 R18.1 50.97,16.13 52.27,16.13 52.65,15.75 J23.2 | 49.69,16.17 49.71,16.15 49.71,13.51 49.1,12.9 46.48,12.9 45.88,12.31 | 45.88,12.31 45.74,12.17 L3.P$1 | J24.1 42.57,13.06 45.14,13.06 45.88,12.31
N$33
  Top 0.254: U6.4 61.21,10.7 L4.2 60.75,10.41 59.44,10.41 59.31,10.29 59.31,8.26 59.69,7.87 60.2,7.87 60.45,7.62 61.8,7.62 C16.P$1
N$34
  Top 0.203: R8.P$2 66.04,7.7 D1.A
N$35
  Top 0.203: U6.7 64.49,7.72 D1.C 64.26,7.24 63.3,7.24 C16.P$2
N$36
  Top 0.406: J22.3 R17.2
N$37
  Top 0.406: J22.2 R18.2
N$38  (via drill 0.33 pad 0.69)
  Top 0.203: U8.4 88.34,8.91 88.29,8.87 | 88.29,8.87 88.23,8.8 | 88.23,8.8 88.19,8.76 C23.P$1 | 88.29,8.87 88.29,8.84 | v88.88,8.46 88.57,8.46 88.23,8.8
  Top 0.406: R24.1 R25.1 89.04,16.15 90.47,16.15 91.26,15.37 J42.2
  Bottom 0.203: 91.31,9.55 91.31,9.6 | 91.31,9.6 J42.2 | v88.88,8.46 90.17,8.46 91.31,9.6
N$39
  Top 0.203: C15.P$2 R7.P$1 65.08,10.85 U6.1
N$40
  Top 0.203: J36.2 71.12,9.65 74.09,6.68 78.03,6.68 78.64,7.29 78.64,8.05 78.54,8.15 U7.8
N$41
  Top 0.254: U7.4 74.55,10.7 L5.2 74.38,10.54 73.74,10.54 72.92,9.73 72.92,8.74 73.86,7.8 75.34,7.8 C20.P$1
N$42
  Top 0.254: D2.A 79.43,8.08 79.5,8.15 R10.P$2
N$43
  Top 0.254: U7.7 78.08,7.64 D2.C 77.67,7.62 77.29,8 C20.P$2
N$44  (via drill 0.33 pad 0.69)
  Top 0.254: U7.1 78.97,10.69 79.3,10.36 R11.P$1 79.5,10.24 v79.83,9.86 | v81.13,8.59 C19.P$2
  Bottom 0.254: v79.83,9.86 79.93,9.78 v81.13,8.59
N$45
  Top 0.406: J34.3 R22.2
N$46
  Top 0.254: R9.P$1 R11.P$2
N$47
  Top 0.406: R19.2 J28.3
N$48
  Top 0.406: R20.2 J28.2
N$49
  Top 0.406: J34.2 R23.2
N$50  (via drill 0.33 pad 0.69)
  Top 0.254: L5.1 74.48,9.17 | 74.48,9.17 74.81,8.84 C18.P$1 76.22,8.85 U7.5 | 74.48,9.17 74.48,8.52 v74.47,8.51
  Top 0.406: J35.2 80.37,15.85 78.94,15.85 78.62,16.17 R23.1 R22.1 74.68,15.88 J36.1
  Bottom 0.254: v74.47,8.51 72.82,8.51 72.52,8.81 72.52,10.92 J36.1
N$51
  Top 0.406: R24.2 J41.3
N$52
  Top 0.203: R12.P$2 86.82,10.13 | 86.82,10.13 R13.P$1 | U8.2 86.82,10.13
N$53
  Top 0.203: U8.1 88.32,10.6 88.32,11.89 87.88,12.32 R14.P$1 87.43,12.04 87.22,11.84 87,11.84 86.87,11.71 86.87,11.48 C22.P$1
N$54  (via drill 0.33 pad 0.69)
  Top 0.203: v87.5,5.89 88.13,5.89 R30.3
  Bottom 0.203: J44.2 86.67,6.73 v87.5,5.89
N$55
  Top 0.406: R25.2 J41.2
N$57
  Top 0.203: J45.2 83.21,14.35 85.24,12.32 R14.P$2
N$58
  Top 0.203: R30.2 86.08,6.94 84.78,8.23 84.78,10.21 J45.1
V_BATT
  Top 0.203: 98.35,15.09 98.35,16.84 97.66,17.53 95.76,17.53 | 95.76,17.53 J1.1 | 95.76,17.53 95.76,19.76 J9.1 | J1.1 94.46,14.12 94.64,13.95 R1.P$2 | B1.+ 94.08,9.5 93.47,10.11 93.47,15.24 J1.1
  Top 0.406: J2.1 12.95,19.56 J3.1 | J10.1 25.04,19.53 J11.1 | J16.1 38.73,19.43 J17.1 | J22.1 53.98,19.56 J23.1 | J28.1 66.93,19.18 J29.1 | J34.1 80.39,19.43 J35.1
  Bottom 0.406: J9.1 94.44,21.06 91.34,24.16 85.01,24.16 83.46,22.61 J34.1 J34.4 J28.1 J28.4 J22.1 J22.4 J16.1 J16.4 J10.1 J10.4 J2.1 J2.4
VCOM
  Top 0.203: U8.3 87.46,9.68 R13.P$2 87.43,9.35 87.3,9.22 86.18,9.22 85.93,8.97 85.93,8 86.39,7.54 90.12,7.54 90.65,7.01 90.65,3.61 90.17,3.12 J40.1

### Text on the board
tPlace: Vbatt | 10 | 100k | 10 | 100k | 10 | 100k | 10 | 100k | 10 | 100k | Vbatt | Vbatt | + | - | Vbatt | Vbatt | Vbatt | Vbatt | 330V/A | IN | 3.3V | 15V | 25V | -15V | -32V | VCOM | 1.8V | VS_CTRL | !SHDN! | Bat. | VSW | CE | !SHDN! | !SHDN! | !SHDN! | GND | GND | GND | GND | GND | GND | - 1.8V + | - 15V + | - 25V + | - -15V + | - -32V + | - VCOM + | - 3.3V +
bPlace: Flexible Smartwatch Power Prototype - Nick Ames 2017 - http://www.fetchmodus.org/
